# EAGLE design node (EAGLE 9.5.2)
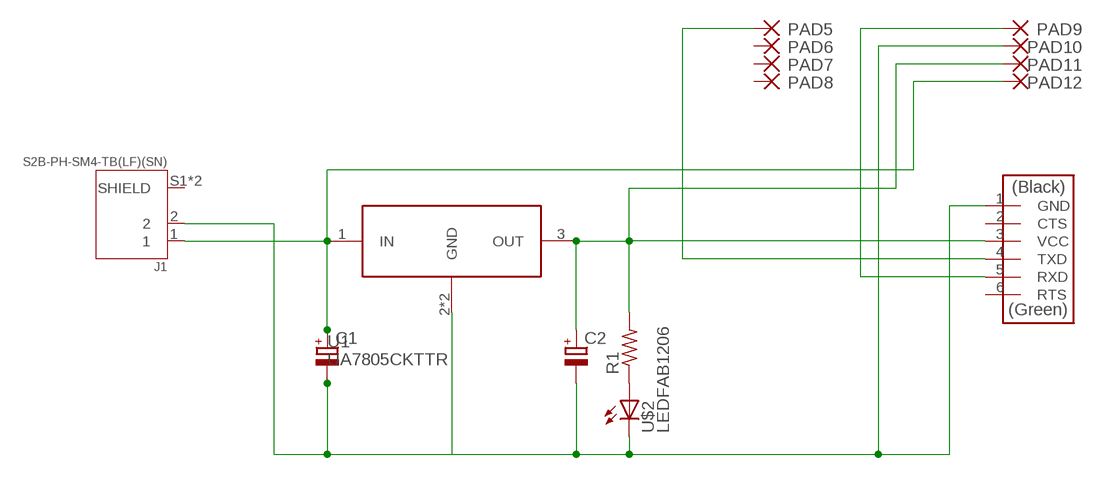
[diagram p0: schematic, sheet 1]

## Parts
C1  CPOL-EUSANYO_SMD_F8  [SANYO-OSCON_SMD_F8]
C2  CPOL-EUSANYO_SMD_F8  [SANYO-OSCON_SMD_F8]
J1  S2B-PH-SM4-TB(LF)(SN)  [JST_S2B-PH-SM4-TB(LF)(SN)]
PAD5  SMD2  [SMD1,27-2,54]
PAD6  SMD2  [SMD1,27-2,54]
PAD7  SMD2  [SMD1,27-2,54]
PAD8  SMD2  [SMD1,27-2,54]
PAD9  SMD2  [SMD1,27-2,54]
PAD10  SMD2  [SMD1,27-2,54]
PAD11  SMD2  [SMD1,27-2,54]
PAD12  SMD2  [SMD1,27-2,54]
R1  R1206FAB  [R1206FAB]
U1  UA7805CKTTR  [TO-263-3]
U$1  CONN_06_FTDI-SMD-HEADER  [1X06SMD]
U$2  LEDFAB1206  [LED1206FAB]

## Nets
N$1: C1.- C2.- J1.2 PAD10.1(P) U1.2(GND) U1.TAB(GND) U$1.1(GND) U$2.2(C)
N$2: R1.1 U$2.1(A)
N$6: PAD5.1(P) U$1.4(TXD)
N$10: C2.+ PAD11.1(P) R1.2 U1.3(OUT) U$1.3(VCC)
N$15: C1.+ J1.1 PAD12.1(P) U1.1(IN)
N$24: PAD9.1(P) U$1.5(RXD)
Unconnected: J1.S1(SHIELD) J1.S2(SHIELD) PAD6.1(P) PAD7.1(P) PAD8.1(P) U$1.2(CTS) U$1.6(RTS)

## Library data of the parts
C1 C2 = rcl-mod:CPOL-EU: POLARIZED CAPACITOR, European symbol; SPICEPREFIX: C
J1 = S2B-PH-SM4-TB_LF__SN_:S2B-PH-SM4-TB(LF)(SN): PH Series 2 Position 2 mm Pitch Surface Mount Side Entry Shrouded Header; DESCRIPTION: Connector Header Surface Mount, Right Angle 2 position 0.079 _2.00mm_; DIGI-KEY_PART_NUMBER: 455-1749-1-ND; DIGIKEY-PURCHASE-URL: https://snapeda.com/shop?store=DigiKey&id=46879; MF: JST Sales; MP: S2B-PH-SM4-TB_LF__SN_; PACKAGE: None
PAD5-PAD12 = wirepad:SMD2: SMD PAD
R1 = fab:R: Resistor (US Symbol)
U1 = UA7805CKTTR:UA7805CKTTR: http://octopart.com/ua7805ckttr-texas+instruments-526009; AVAILABILITY: Unavailable; DESCRIPTION: Linear Voltage Regulator IC 1 Output 1.5A DDPAK/TO-263-3; MF: Texas Instruments; MP: UA7805CKTTR; PACKAGE: TO-263-3 Texas Instruments; PRICE: None
U$1 = fab:CONN_06_FTDI-SMD-HEADER
U$2 = fab:LED: LED

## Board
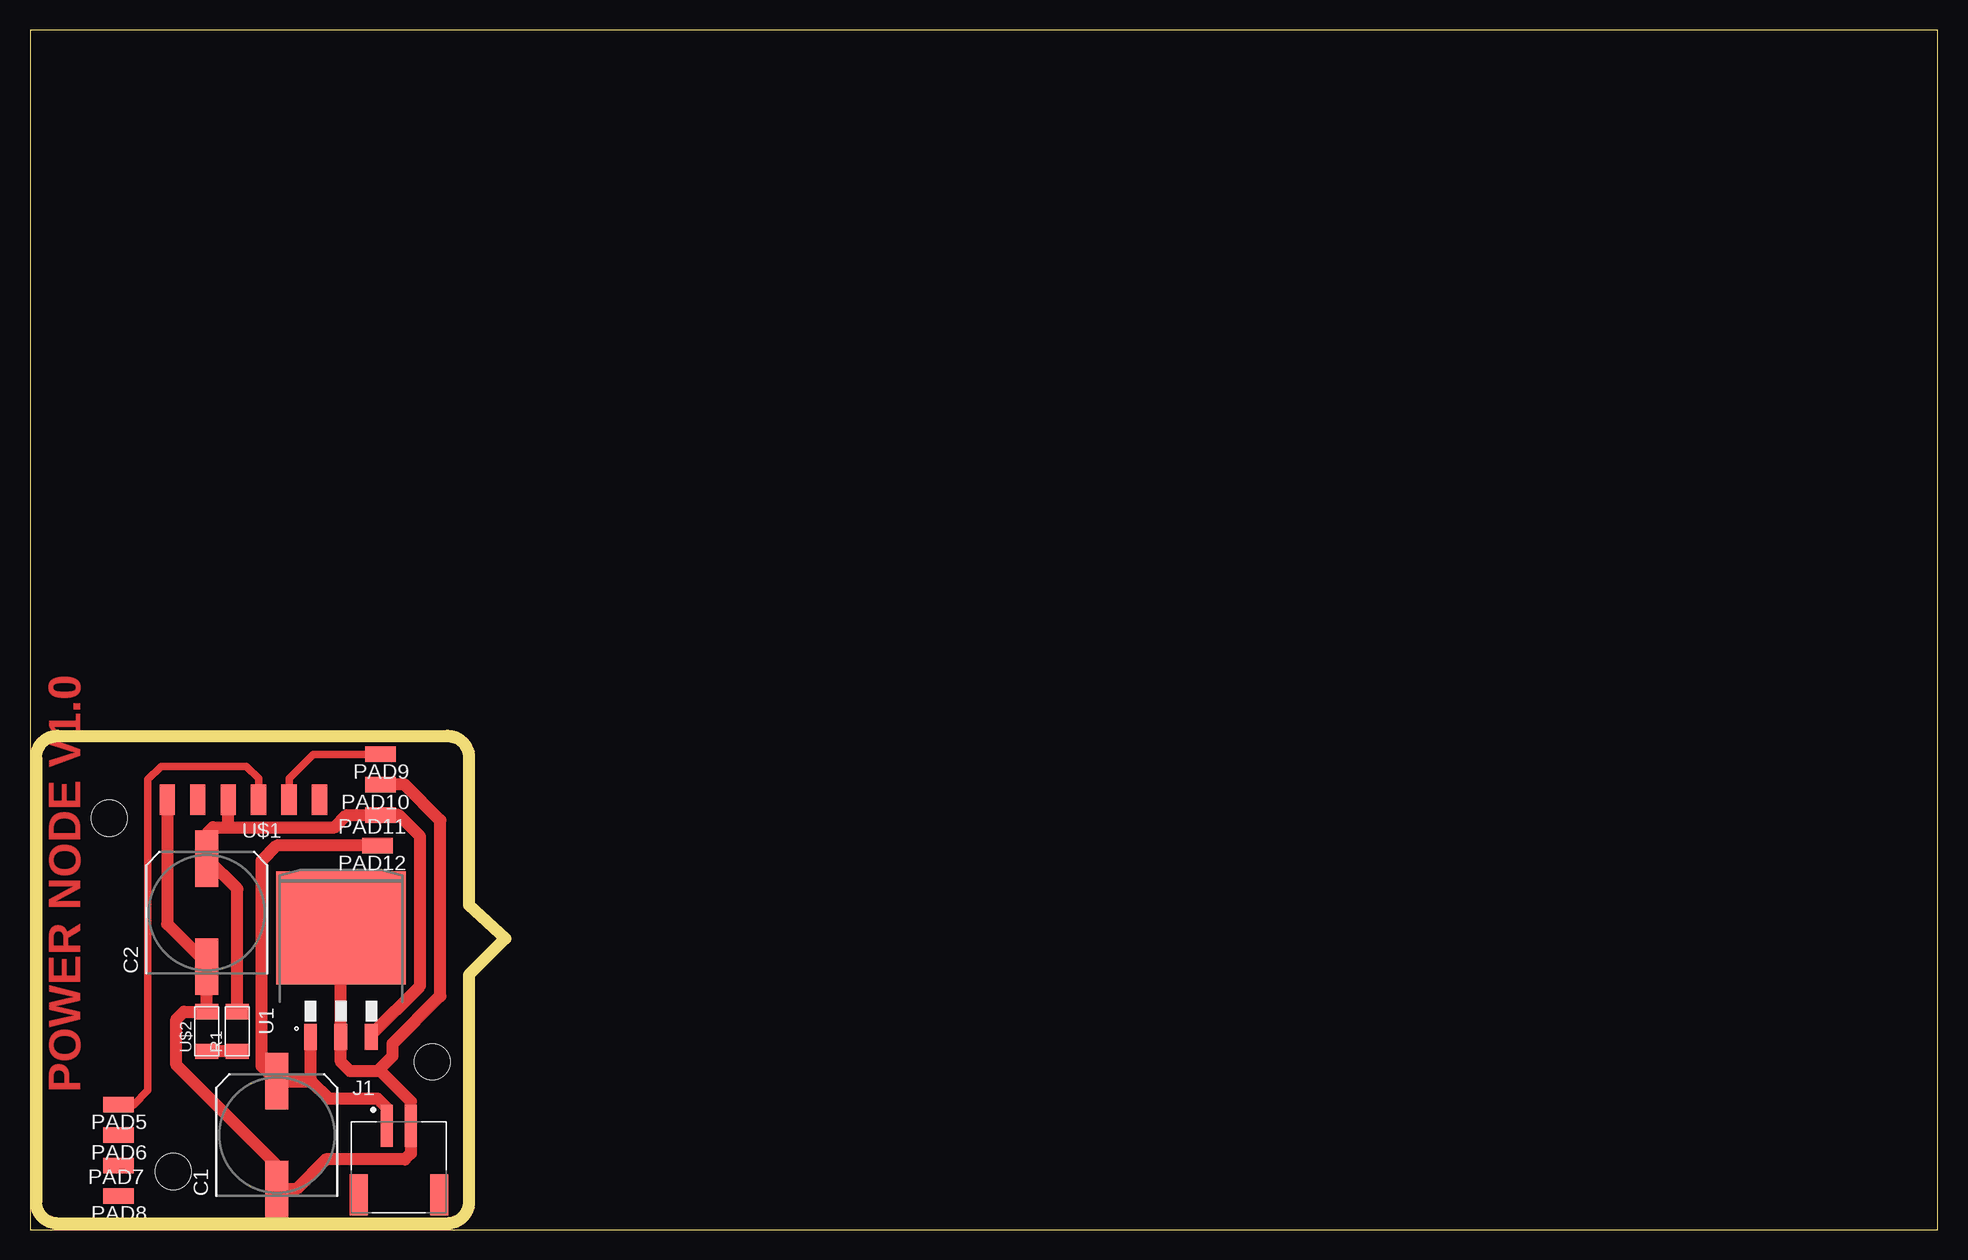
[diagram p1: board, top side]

Size 158.98 x 100 mm. Coordinates in mm from the lower left corner, seen from the top.
Outline: 0,0 158.98,0 158.98,100 0,100 0,0
Copper layers (1*16): Top 0.035mm / dielectric 1.5mm / Bottom 0.035mm
Design rules "default *": minimum track width 6mil, minimum drill 0.35mm, track to track 16mil, track to pad 16mil, pad to pad 16mil, via to via 16mil, smd to smd 16mil, copper to edge 40mil, drill to drill 6mil, minimum pad ring 10mil, minimum via ring 8mil, stop-mask expansion 4mil, vias tented up to drill 0mil, thermal gap 10mil
Holes 3 mm at 11.94,4.83 6.6,34.29 33.53,13.97
Milling: 11 lines

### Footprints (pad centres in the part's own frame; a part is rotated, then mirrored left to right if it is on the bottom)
SANYO-OSCON_SMD_F8 = smd 4.7 x 1.9: + 4.5,0; - -4.5,0
JST_S2B-PH-SM4-TB(LF)(SN) = smd 1 x 3.5: 1 -1,0; 2 1,0 | smd 1.5 x 3.4: S1 -3.35,-5.75; S2 3.35,-5.75
SMD1,27-2,54 = smd 1.27 x 2.54: 1 0,0
R1206FAB = smd 1.27 x 1.905: 1 -1.651,0; 2 1.651,0
TO-263-3 = smd 2.159 x 1.067: 1 -3.251,2.54; 2 -3.251,0; 3 -3.251,-2.54 | smd 9.398 x 10.8: TAB 5.842,0
1X06SMD = smd 2.54 x 1.27: 1 0,6.35; 2 0,3.81; 3 0,1.27; 4 0,-1.27; 5 0,-3.81; 6 0,-6.35
LED1206FAB = smd 1.27 x 1.905: 1 -1.651,0; 2 1.651,0

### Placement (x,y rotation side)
C1  20.57,7.87 90 top
C2  14.73,26.42 90 top
J1  30.73,8.64 0 top
PAD5  7.37,10.41 90 top
PAD6  7.37,7.87 90 top
PAD7  7.37,5.33 90 top
PAD8  7.37,2.79 90 top
PAD9  29.21,39.62 90 top
PAD10  29.21,37.08 90 top
PAD11  29.21,34.54 90 top
PAD12  28.96,32 90 top
R1  17.27,16.51 90 top
U1  25.91,19.3 90 top
U$1  17.78,35.81 90 top
U$2  14.73,16.51 90 top

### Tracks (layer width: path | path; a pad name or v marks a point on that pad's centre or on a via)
N$1
  Top 1.016: PAD10.1 31.24,37.08 34.2,34.12 34.2,19.47 30.23,15.49 30.23,14.48 29.21,13.46 29.21,13.21 | U$1.1 11.43,25.47 14.73,22.17 C2.- U$2.2 12.83,18.16 12.19,17.53 12.19,13.72 20.57,5.33 C1.- 22.17,3.37 24.64,5.84 31.24,5.84 31.73,6.33 J1.2 31.73,10.68 29.21,13.21 | U1.TAB U1.2 25.91,13.97 26.67,13.21 29.21,13.21
N$2
  Top 1.016: R1.1 U$2.1
N$6
  Top 0.61: U$1.4 19.05,37.59 18.03,38.61 10.92,38.61 9.83,37.52 9.83,11.61 8.64,10.41 PAD5.1
N$10
  Top 1.016: U1.3 28.45,16.26 32.51,20.32 32.51,32.77 30.73,34.54 PAD11.1 26.42,34.54 25.4,33.53 16.51,33.53 | 16.51,33.53 15.24,33.53 14.73,33.02 C2.+ 17.27,28.38 R1.2 | 16.51,33.53 U$1.3
N$15
  Top 1.016: U1.1 23.37,12.45 23.44,12.37 | 23.44,12.37 24.89,10.92 28.96,10.92 29.73,10.14 J1.1 | PAD12.1 20.57,32 19.3,30.73 19.3,13.64 C1.+ 23.44,12.37
N$24
  Top 0.61: U$1.5 21.59,37.59 23.62,39.62 PAD9.1

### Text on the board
Top: POWER NODE V1.0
